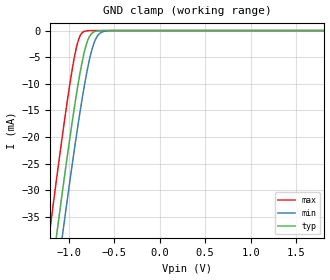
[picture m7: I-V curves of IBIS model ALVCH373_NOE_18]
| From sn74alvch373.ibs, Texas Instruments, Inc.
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[Model]   ALVCH373_NOE_18
Model_type  Input
Vinl=0.5775
Vinh=1.2675
| variable   typ   min   max
C_comp   3.72pF   3.30pF   4.42pF
[Temperature Range]   40   100   -40
| Ambient temperature   25   85   -40
[Voltage range]   1.8   1.65   1.95
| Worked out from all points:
|   GND clamp passes 1 mA (typ) near -0.77 V on its own axis
[GND Clamp]
| ALVCH373_NOE_18
|   Voltage   I(typ)   I(min)   I(max)
-1.8V     -129.8mA   -137.8mA   -119.7mA
-1.205V   -48.27mA   -56.56mA   -37.63mA
-1.125V   -37.77mA   -46.06mA   -27.13mA
-1.06V    -29.44mA   -37.69mA   -18.89mA
-980mV    -19.61mA   -27.69mA   -9.485mA
-925mV    -13.29mA   -21.11mA   -4.122mA
-880mV    -8.606mA   -15.99mA   -1.263mA
-835mV    -4.656mA   -11.25mA   -214.1uA
-780mV    -1.472mA   -6.227mA   -17.15uA
-725mV    -285.9uA   -2.596mA   -1.294uA
-615mV    -6.479uA   -167.8uA   -7.305nA
1.8V      3.326pA    6.142pA    3.026pA
